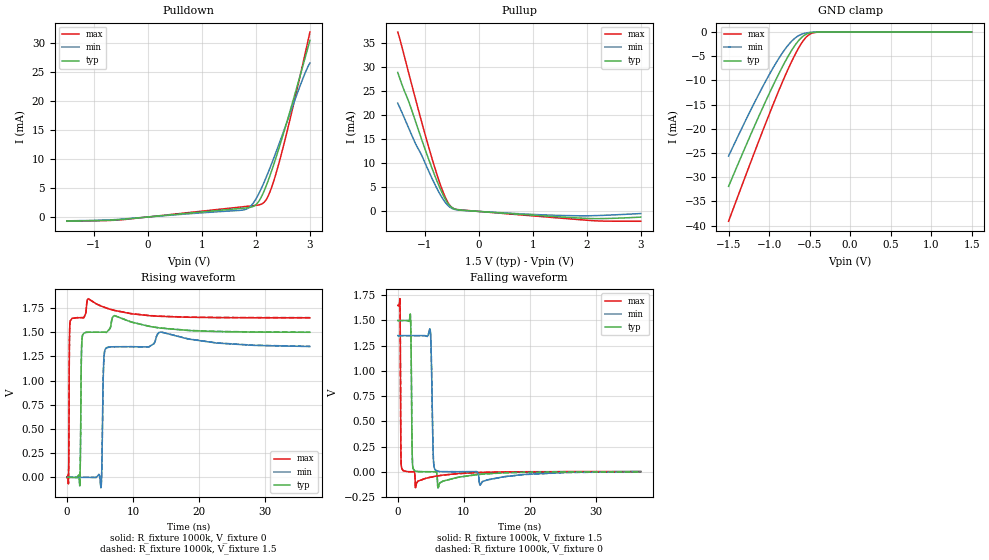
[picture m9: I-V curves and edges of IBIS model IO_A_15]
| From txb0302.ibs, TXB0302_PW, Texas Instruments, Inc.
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[Model]   IO_A_15
Model_type  3-state
Enable   Active-High
Vref =   0
Rref =   1000k
Cref =   50p
Vmeas =   0.75
| variable   typ   min   max
C_comp   3.43pF   3.22pF   3.60pF
| C_pullup   3.67pF   3.28pF   3.86pF
| C_pulldown   3.66pF   3.28pF   3.85pF
| C_tri-state   3.43pF   3.22pF   3.60pF
[Temperature Range]   40   100   -40
| Ambient temperature   25   85   -40
[Voltage range]   1.5   1.35   1.65
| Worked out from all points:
|   slope of the pulldown table from 0 to 0.225 V, typ, clamps not added: 1.13 kohm
|   slope of the pullup table from 0 to 0.225 V, typ, clamps not added: 1.26 kohm
|   GND clamp passes 1 mA (typ) near -0.59 V on its own axis
|   rising waveform, R_fixture 1000k, V_fixture 0: 20-80 % time 127ps typ, 189ps min, 75ps max; typ from 0 V to 1.5 V
|   falling waveform, R_fixture 1000k, V_fixture 1.5: 20-80 % time 135ps typ, 230ps min, 74.3ps max; typ from 1.5 V to 0.002 V
|   rising waveform, R_fixture 1000k, V_fixture 1.5: 20-80 % time 127ps typ, 189ps min, 75ps max; typ from 0.002 V to 1.5 V
|   falling waveform, R_fixture 1000k, V_fixture 0: 20-80 % time 135ps typ, 230ps min, 74.3ps max; typ from 1.5 V to 0 V
[GND Clamp]
| IO_A_15
|   Voltage   I(typ)   I(min)   I(max)
-1.5V     -31.88mA   -25.62mA   -39.1mA
-1.3V     -24.01mA   -18.61mA   -30.13mA
-1.13V    -17.53mA   -12.93mA   -22.64mA
-985mV    -12.24mA   -8.412mA   -16.42mA
-865mV    -8.125mA   -5.054mA   -11.49mA
-760mV    -4.86mA    -2.616mA   -7.464mA
-665mV    -2.391mA   -1.068mA   -4.201mA
-585mV    -926.4uA   -370.4uA   -1.947mA
-515mV    -268.3uA   -112.4uA   -649.1uA
-455mV    -68.84uA   -31.05uA   -160.1uA
-365mV    -6.097uA   -3.221uA   -9.086uA
1.5V      240.8pA    68.49nA    22.97pA
[Pulldown]
| IO_A_15
|   Voltage   I(typ)   I(min)   I(max)
-1.5V     -706.8uA   -664.3uA   -741.6uA
-500mV    -439.1uA   -380.5uA   -495.2uA
1.77V     1.522mA    1.224mA    1.777mA
1.885V    1.648mA    1.724mA    1.891mA
1.99V     2.048mA    2.965mA    1.998mA
2.135V    4.149mA    5.662mA    2.409mA
2.195V    5.507mA    6.977mA    3.078mA
2.26V     7.161mA    8.483mA    4.358mA
2.425V    11.85mA    12.55mA    9.266mA
2.66V     19.22mA    18.64mA    18.01mA
2.88V     26.49mA    24.18mA    26.95mA
3V        30.54mA    26.63mA    31.97mA
[Pullup]
| IO_A_15
|   Voltage   I(typ)   I(min)   I(max)
-1.5V     28.9mA     22.51mA    37.31mA
-1.18V    19.02mA    14.31mA    23.75mA
-1.05V    14.73mA    11.5mA     18.31mA
-815mV    7.49mA     5.679mA    9.129mA
-715mV    4.766mA    3.535mA    5.692mA
-630mV    2.774mA    2.033mA    3.203mA
-560mV    1.516mA    1.128mA    1.656mA
-495mV    784.1uA    617.3uA    810.4uA
-320mV    263uA      225.3uA    302.8uA
1.47V     -1.115mA   -826.1uA   -1.356mA
2.16V     -1.494mA   -872.2uA   -1.956mA
3V        -1.19mA    -441.5uA   -2.05mA
[Ramp]
| IO_A_15
| variable   typ   min   max
dV/dt_r   1.06/1.76E-10   0.97/2.67E-10   1.15/1.09E-10
dV/dt_f   1.03/1.74E-10   0.93/2.92E-10   1.12/9.62E-11
R_load = 1000k
[Rising Waveform]
| IO_A_15
R_fixture =   1000k
C_fixture =   0
L_fixture =   0
V_fixture =   0
V_fixture_min = 0
V_fixture_max = 0
|   Time   V(typ)   V(min)   V(max)
0s        385.6nV    2.056uV    45.7nV
237ps     257.2nV    2.056uV    -33.29mV
477ps     489.9nV    2.056uV    1.605V
1.941ns   -88.28mV   1.877uV    1.65V
2.253ns   1.395V     1.724uV    1.65V
3.213ns   1.499V     -69.74uV   1.846V
5.165ns   1.5V       -103.6mV   1.77V
5.565ns   1.5V       1.183V     1.759V
6.005ns   1.498V     1.339V     1.748V
36.79ns   1.499V     1.352V     1.648V
[Falling Waveform]
| IO_A_15
R_fixture =   1000k
C_fixture =   0
L_fixture =   0
V_fixture =   1.5
V_fixture_min = 1.35
V_fixture_max = 1.65
|   Time   V(typ)   V(min)   V(max)
0s        1.5V       1.35V      1.65V
333ps     1.5V       1.35V      1.675V
525ps     1.5V       1.35V      64.53mV
1.901ns   1.564V     1.35V      212.9uV
2.221ns   99.98mV    1.35V      121.1uV
2.685ns   6.496mV    1.35V      -159.5mV
4.925ns   112.1uV    1.4V       -54.75mV
5.389ns   73.52uV    138.6mV    -48.48mV
5.821ns   -958.5uV   11.73mV    -43.28mV
36.79ns   1.6mV      1.026mV    1.614mV
[Rising Waveform]
| IO_A_15
R_fixture =   1000k
C_fixture =   0
L_fixture =   0
V_fixture =   1.5
V_fixture_min = 1.35
V_fixture_max = 1.65
|   Time   V(typ)   V(min)   V(max)
0s        1.69mV     1.782mV    1.625mV
237ps     1.69mV     1.782mV    -31.68mV
477ps     1.69mV     1.782mV    1.606V
1.941ns   -86.56mV   1.782mV    1.65V
2.253ns   1.395V     1.781mV    1.65V
3.213ns   1.499V     1.71mV     1.847V
5.165ns   1.5V       -101.7mV   1.77V
5.565ns   1.5V       1.184V     1.76V
6.005ns   1.498V     1.339V     1.749V
36.79ns   1.5V       1.354V     1.65V
[Falling Waveform]
| IO_A_15
R_fixture =   1000k
C_fixture =   0
L_fixture =   0
V_fixture =   0
V_fixture_min = 0
V_fixture_max = 0
|   Time   V(typ)   V(min)   V(max)
0s        1.498V     1.348V     1.648V
333ps     1.498V     1.348V     1.674V
525ps     1.498V     1.348V     64.4mV
1.901ns   1.562V     1.348V     179.4uV
2.221ns   99.63mV    1.348V     87.67uV
2.685ns   6.452mV    1.348V     -159.6mV
4.925ns   77.81uV    1.398V     -55.52mV
5.389ns   39.26uV    138mV      -49.35mV
5.821ns   -1.006mV   11.67mV    -44.23mV
36.79ns   -86.27uV   -732.9uV   -9.807uV
